PROGRAM MAIN
VAR	
	//Outputs to the Box
		iControlWord AT%Q*:UINT;
		iModesOfOperation AT%Q*:SINT;
		iTargetPosition AT%Q*:DINT;
		iMotorDriveSubmodeSelect AT%Q*:UDINT;
	//Inputs from the Box
		iStatusWord AT%I*:UINT;	
		iModesOfOperationDisplay AT%I*:SINT;	
		iActualPosition AT%I*:DINT;	
	//Program-variables 	
		bStart : BOOL;		//Starts to move the motor between the positions 0 and 10000
		iStep : USINT :=0 ;	//"State-Machine" for the program
		
END_VAR


IF(bStart AND (iStep = 0)) THEN	
iModesOfOperation := 1;
iMotorDriveSubmodeSelect :=1;
iControlWord :=6;
iStep := 1;	
END_IF

IF(NOT bStart AND (iStep > 0)) THEN	
iControlWord :=0;
iStep := 0;	
END_IF

IF((iStep = 1)AND((iStatusWord AND 16#EF)=16#21)) THEN	
iControlWord :=7;
iStep := 2;	
END_IF

IF((iStep = 2)AND((iStatusWord AND 16#EF)=16#23)) THEN	
iControlWord :=15;
iStep := 3;	
END_IF

IF((iStep = 3)AND((iStatusWord AND 16#EF)=16#27)) THEN	
iTargetPosition := 0;	
iControlWord :=31;
iStep := 4;	
END_IF

IF((iStep = 4)AND((iStatusWord AND 16#1000)=16#1000)) THEN	
iControlWord :=15;
iStep := 5;
END_IF

IF((iStep = 5)AND((iStatusWord AND 16#400)=16#400)) THEN		
iTargetPosition := 10000;	
iControlWord :=31;
iStep := 6;	
END_IF

IF((iStep = 6)AND((iStatusWord AND 16#1000)=16#1000)) THEN	
iControlWord :=15;
iStep := 7;
END_IF

IF((iStep = 7)AND((iStatusWord AND 16#400)=16#400)) THEN	
iTargetPosition := 0;
iControlWord :=31;
iStep := 4;
END_IF

END_PROGRAM
